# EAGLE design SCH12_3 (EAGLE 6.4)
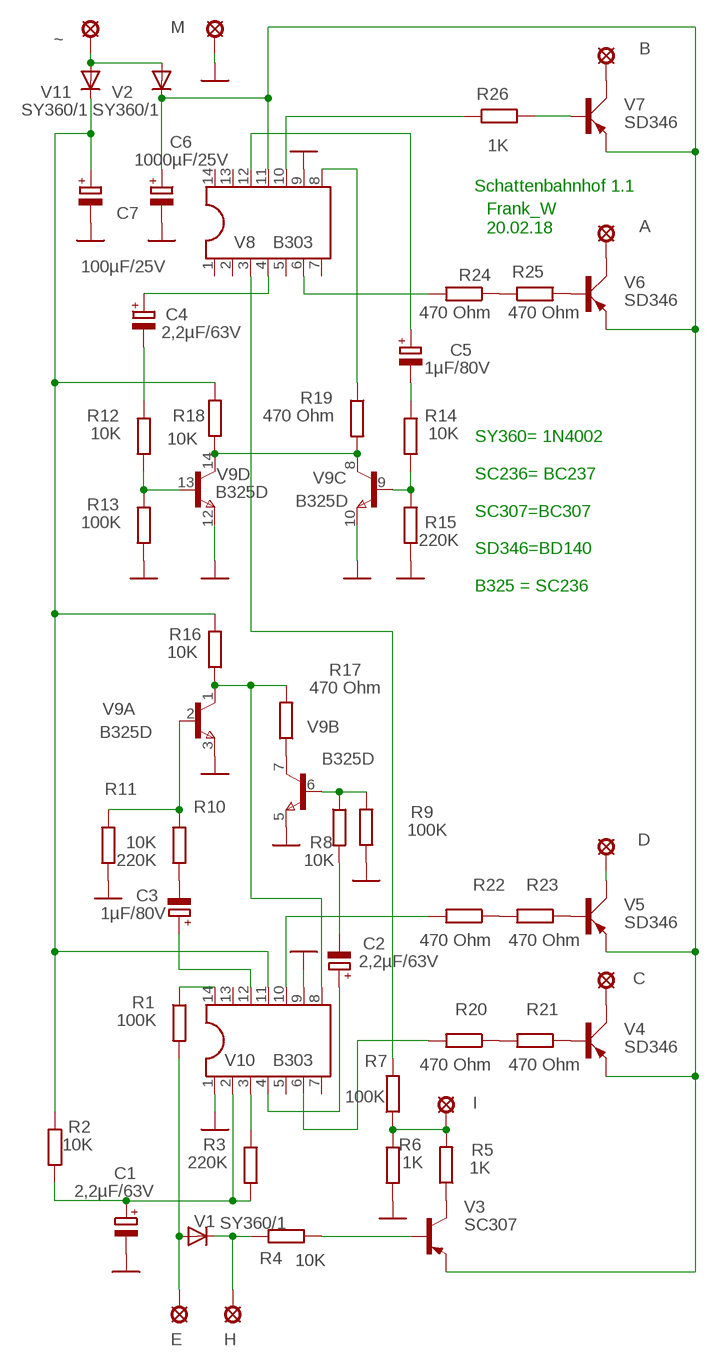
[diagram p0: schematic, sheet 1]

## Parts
A  LSP10  [LSP10]
B  LSP10  [LSP10]
C  LSP10  [LSP10]
C1  2,2µF/63V  CPOL-EUE5-5  [E5-5]
C2  2,2µF/63V  CPOL-EUE5-5  [E5-5]
C3  1µF/80V  CPOL-EUE2-5  [E2-5]
C4  2,2µF/63V  CPOL-EUE2-5  [E2-5]
C5  1µF/80V  CPOL-EUE5-5  [E5-5]
C6  1000µF/25V  CPOL-EUE22-9AXIAL  [E22-9]
C7  100µF/25V  CPOL-EUE2.5-6  [E2,5-6]
D  LSP10  [LSP10]
E  LSP10  [LSP10]
H  LSP10  [LSP10]
I  LSP10  [LSP10]
M  LSP10  [LSP10]
R1  100K  R-EU_0207/12  [0207/12]
R2  10K  R-EU_0207/12  [0207/12]
R3  220K  R-EU_0207/12  [0207/12]
R4  10K  R-EU_0207/12  [0207/12]
R5  1K  R-EU_0207/12  [0207/12]
R6  1K  R-EU_0207/12  [0207/12]
R7  100K  R-EU_0207/12  [0207/12]
R8  10K  R-EU_0207/12  [0207/12]
R9  100K  R-EU_0207/12  [0207/12]
R10  10K  R-EU_0207/12  [0207/12]
R11  220K  R-EU_0207/12  [0207/12]
R12  10K  R-EU_0207/12  [0207/12]
R13  100K  R-EU_0207/12  [0207/12]
R14  10K  R-EU_0207/12  [0207/12]
R15  220K  R-EU_0207/12  [0207/12]
R16  10K  R-EU_0207/12  [0207/12]
R17  470 Ohm  R-EU_0207/12  [0207/12]
R18  10K  R-EU_0207/12  [0207/12]
R19  470 Ohm  R-EU_0207/12  [0207/12]
R20  470 Ohm  R-EU_0207/12  [0207/12]
R21  470 Ohm  R-EU_0207/12  [0207/12]
R22  470 Ohm  R-EU_0207/12  [0207/12]
R23  470 Ohm  R-EU_0207/12  [0207/12]
R24  470 Ohm  R-EU_0207/12  [0207/12]
R25  470 Ohm  R-EU_0207/10  [0207/10]
R26  1K  R-EU_0207/10  [0207/10]
V1  SY360/1  1N4004  [DO41-10]
V2  SY360/1  1N4004  [DO41-10]
V3  SC307  BC448  [TO92-EBC]
V4  SD346  BD140  [TO126AV]
V5  SD346  BD140  [TO126AV]
V6  SD346  BD140  [TO126AV]
V7  SD346  BD140  [TO126AV]
V8  B303  DIL14  [DIL14]
V9  B325D  MAT-04Y  [DIL14]
V10  B303  DIL14  [DIL14]
V11  SY360/1  1N4004  [DO41-10]
~  LSP10  [LSP10]

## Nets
GND: C1.- C6.- C7.- M.MP R6.2 R9.1 R11.2 R13.2 R15.2 V8.9 V9.3(A:E) V9.5(B:E) V9.10(C:E) V9.12(D:E) V10.1 V10.9
N$1: V2.A V11.A ~.MP
N$2: B.MP V7.C
N$3: A.MP V6.C
N$4: R17.1 V9.7(B:C)
N$5: R25.2 V6.B
N$6: R26.2 V7.B
N$7: R19.1 V8.8
N$8: C5.+ V8.12
N$9: C5.- R14.1
N$10: R26.1 V8.10
N$11: R24.1 R25.1
N$13: C7.+ R2.1 R16.2 R18.2 V10.11 V11.C
N$14: R16.1 R17.2 V9.1(A:C) V10.8
N$15: C4.+ V8.4
N$16: C4.- R12.1
N$17: R24.2 V8.6
N$18: E.MP R1.2 V1.A
N$19: R1.1 V10.14
N$20: H.MP R4.2 V1.C
N$21: I.MP R5.2 R6.1 R7.1
N$22: R4.1 V3.B
N$23: R5.1 V3.C
N$24: C6.+ V2.C V3.E V4.E V5.E V6.E V7.E V8.11
N$25: C.MP V4.C
N$26: D.MP V5.C
N$27: R21.1 V4.B
N$28: R23.1 V5.B
N$29: C1.+ R2.2 R3.2 V10.2
N$30: C2.+ V10.4
N$31: R3.1 V10.3
N$32: C2.- R8.2
N$33: R20.2 V10.6
N$34: R8.1 R9.2 V9.6(B:B)
N$35: C3.- R10.2
N$36: C3.+ V10.12
N$37: R22.2 V10.10
N$39: R10.1 R11.1 V9.2(A:B)
N$40: R12.2 R13.1 V9.13(D:B)
N$41: R18.1 R19.2 V9.8(C:C) V9.14(D:C)
N$42: R14.2 R15.1 V9.9(C:B)
N$43: R20.1 R21.2
N$44: R22.1 R23.2
N$46: R7.2 V8.3
Unconnected: V8.1 V8.2 V8.5 V8.7 V8.13 V8.14 V10.5 V10.7 V10.13

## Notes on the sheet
- Schattenbahnhof 1.1
- Frank_W
  20.02.18
- SY360= 1N4002
  
  SC236= BC237
  
  SC307=BC307
  
  SD346=BD140
  
  B325 = SC236

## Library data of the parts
A B C D E H I M ~ = solpad:LSP10: SOLDER PAD
C1-C7 = rcl:CPOL-EU: POLARIZED CAPACITOR, European symbol
R1-R26 = rcl:R-EU_: RESISTOR, European symbol
V1 V2 V11 = diode:1N4004: DIODE
V3 = transistor-pnp:BC448*: PNP Transistror
V4-V7 = transistor-power:BD140: PNP TRANSISTOR
V8 V10 = ic-package:DIL14: Dual In Line / Socket
V9 = linear:MAT-04: Quad TRANSISTOR

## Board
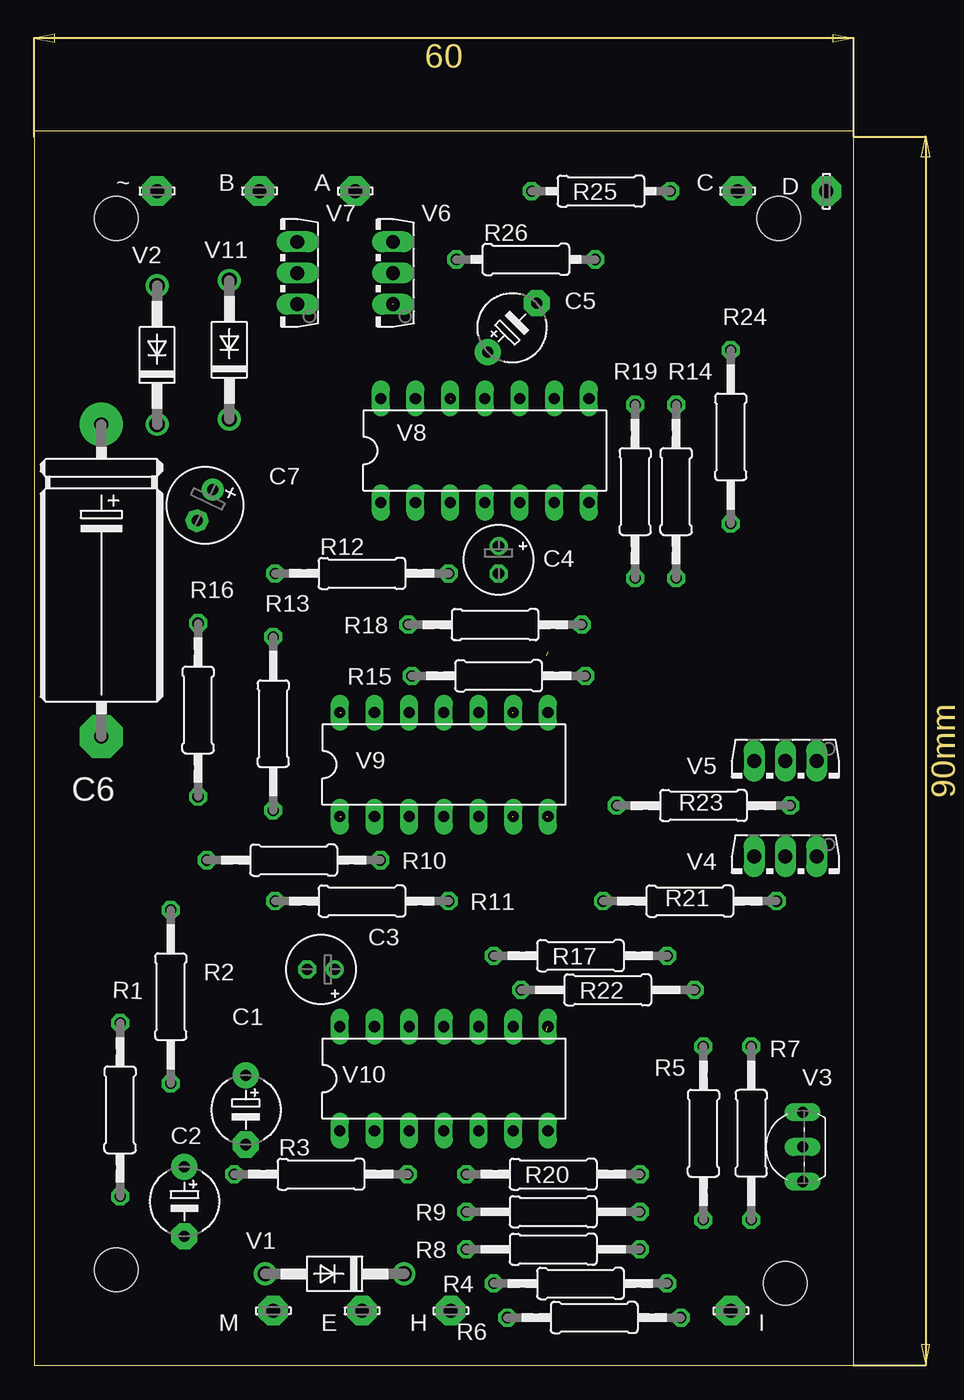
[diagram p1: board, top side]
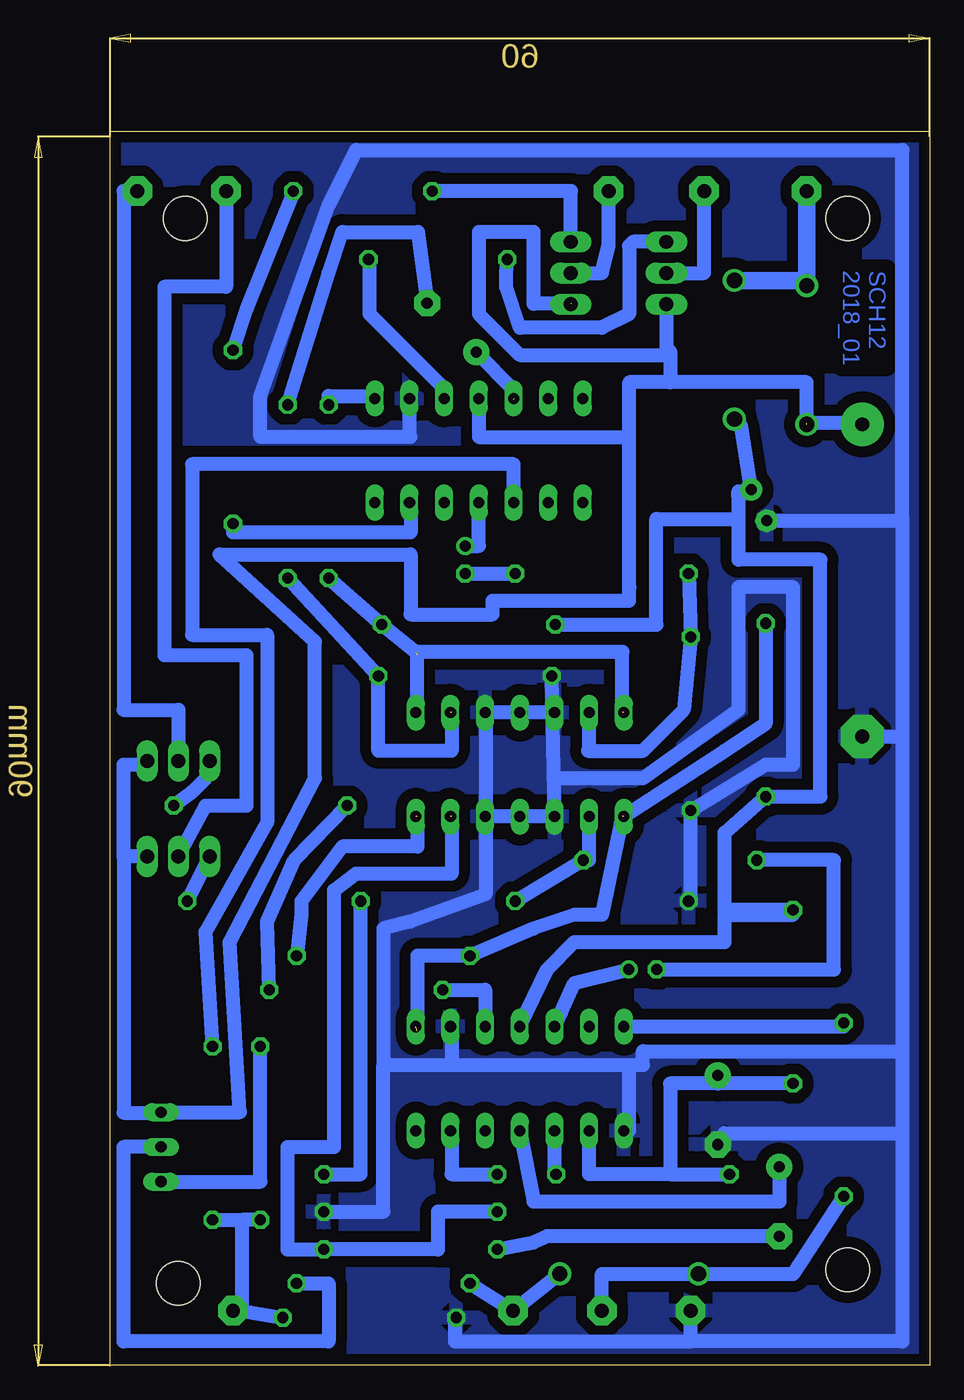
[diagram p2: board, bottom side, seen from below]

Size 65.56 x 97.5 mm. Coordinates in mm from the lower left corner, seen from the top.
Outline: 0,90.4 0,0 60,0 60,90.4 0,90.4
Copper layers (1*16): Top 0.035mm / dielectric 1.5mm / Bottom 0.035mm
Design rules "default *": minimum track width 20mil, minimum drill 24mil, track to track 8mil, track to pad 8mil, pad to pad 8mil, via to via 8mil, smd to smd 8mil, copper to edge 20mil, drill to drill 8mil, minimum pad ring 10mil, minimum via ring 8mil, stop-mask expansion 4mil, vias tented up to drill 0mil, thermal gap 20mil
Holes 3.2 mm at 55,6 6,7 6,84 54.5,84

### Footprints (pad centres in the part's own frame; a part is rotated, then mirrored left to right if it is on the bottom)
LSP10 = drill 1.016 pad 2.159 octagon: MP 0,0
E5-5 = drill 0.813 pad 1.905: + -2.54,0 | drill 0.813 pad 1.905 octagon: - 2.54,0
E2-5 = drill 0.813 pad 1.27: + -1.016,0 | drill 0.813 pad 1.27 octagon: - 1.016,0
E22-9 = drill 1.016 pad 3.15: + -11.43,0 | drill 1.016 pad 3.15 octagon: - 11.43,0
E2,5-6 = drill 0.813 pad 1.6: + -1.27,0 | drill 0.813 pad 1.6 octagon: - 1.27,0
0207/12 = drill 0.813 octagon: 1 -6.35,0; 2 6.35,0
0207/10 = drill 0.813 octagon: 1 -5.08,0; 2 5.08,0
DO41-10 = drill 1.118: A 5.08,0; C -5.08,0
TO92-EBC = drill 0.813 long: B 0,-1.27; C -2.54,-1.27; E 2.54,-1.27
TO126AV = drill 1.016 long: B 2.286,-1.27; C 0,-1.27; E -2.286,-1.27
DIL14 = drill 0.813 long: 1 -7.62,-3.81; 2 -5.08,-3.81; 3 -2.54,-3.81; 4 0,-3.81; 5 2.54,-3.81; 6 5.08,-3.81; 7 7.62,-3.81; 8 7.62,3.81; 9 5.08,3.81; 10 2.54,3.81; 11 0,3.81; 12 -2.54,3.81; 13 -5.08,3.81; 14 -7.62,3.81

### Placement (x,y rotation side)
A  23.5,86 0 top
B  16.5,86 0 top
C  51.5,86 0 top
C1  15.5,18.71 270 top
C2  11,12 270 top
C3  21,29 180 top
C4  34,59 270 top
C5  35,76 45 top
C6  4.92,57.49 270 top
C7  12.5,63 243.5 top
D  58,86 90 top
E  24,4 0 top
H  30.5,4 0 top
I  51,4 0 top
M  17.5,4 0 top
R1  6.29,18.72 270 top
R2  10,27 270 top
R3  21,14 180 top
R4  40,6 180 top
R5  49,17 270 top
R6  41,3.5 180 top
R7  52.5,17 90 top
R8  38,8.5 180 top
R9  38,11.25 180 top
R10  19,37 180 top
R11  24,34 180 top
R12  24,58 180 top
R13  17.5,47 270 top
R14  47,64 270 top
R15  34,50.5 180 top
R16  12,48 270 top
R17  40,30 180 top
R18  33.75,54.25 180 top
R19  44,64 270 top
R20  38,14 180 top
R21  48,34 180 top
R22  42,27.5 180 top
R23  49,41 180 top
R24  51,68 270 top
R25  41.5,86 180 top
R26  36,81 180 top
V1  22,6.7 180 top
V2  9,74 90 top
V3  55,16 90 top
V4  55,36 180 top
V5  55,43 180 top
V6  25,80 90 top
V7  18,80 90 top
V8  33,67 0 top
V9  30,44 0 top
V10  30,21 0 top
V11  14.29,74.38 90 top
~  9,86 0 top

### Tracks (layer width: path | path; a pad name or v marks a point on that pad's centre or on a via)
GND
  Bottom 1.016: C7.- 2,61.86 2,46.06 | 2,62 2,89 42,89 44,85 49,71 49,68 38,68 38.08,68.08 V8.9 | 2,46.06 2,23 | 2,23 2,17 | 2,17 2,1.75 17.5,1.75 | 17.5,1.75 M.MP | C1.- 15,16.17 15,17 2,17 | C6.- 2,46.06 | 34.75,3.5 34.75,1.75 17.5,1.75 | V10.9 35,24.81 35,22 | 35,22 22,22 | 22,22 21,22 21,23 2,23 | R9.1 40,11.25 40,22 | 40,22 35,22 | 32.5,47.81 32.5,40.19 | 32.5,40.19 32.5,34.5 38,32.5 40,32 40,22 | 27.46,43 21,43 14,48 14,57 10,57 10,44 12,44 R13.2 17.5,34 R11.2 | V10.1 22,17.19 22,22 | R15.2 V9.3 32.5,40.19 | V9.12 V9.10 | 32.5,40.19 V9.5
  pour Bottom (isolate 0.813): 0,90 60,90 60,0 0,0
N$1
  Bottom 1.27: V11.A 9,79.46 V2.A ~.MP
N$2
  Bottom 1.016: V7.C 16.5,80 B.MP
N$3
  Bottom 1.016: V6.C 24,80 23.5,82 A.MP
N$4  (1 unrouted)
  Bottom 1.016: 37.5,40.19 37.5,38 43,38 46,34 46,33 R17.1
N$5
  Bottom 1.016: V6.B 26.27,86 R25.2
N$6
  Bottom 1.016: V7.B 21.71,82.29 22,82 22,77 24,76 30,76 31,79 31,80 R26.2
N$7
  Bottom 1.016: R19.1 44,71 40.81,71 V8.8
N$8  (1 unrouted)
  Bottom 1.016: C5.+ 30.5,71.46 30.5,70.75
N$9
  Bottom 1.016: R14.1 44,80 43,83 37.46,83 C5.-
N$10
  Bottom 1.016: V8.10 35.54,71.54 41,77 41,81 R26.1
N$11
  Bottom 1.016: R24.1 50,77.35 46.5,86 R25.1
N$13
  Bottom 1.016: V11.C 13.79,68.8 C7.+ 14,63.59 | 14,63.59 14,64 | 14,63.59 14,62 | 14,62 14,59 8,59 8,41.65 R16.2 15,39 15,33.35 R2.1 10,33 15,33 15,31 26,31 28,29 V10.11 | R18.2 20,54.25 20,62 14,62
N$14  (2 unrouted)
  Bottom 1.016: 22.5,40.19 24,33 26,33 29,32 R17.2 37.5,30 37.5,24.5 | R16.1 12,47 15,45 V9.1
N$15
  Bottom 1.016: C4.+ 33,60.02 V8.4
N$16
  Bottom 1.016: C4.- 30.35,57.98 R12.1
N$17
  Bottom 1.016: V8.6 38,63.19 38,61 51,61 R24.2
N$18
  Bottom 1.016: E.MP 24,6.7 V1.A 10,6.7 R1.2
N$19
  Bottom 1.016: V10.14 6.29,24.81 R1.1
N$20
  Bottom 1.016: V1.C H.MP R4.2
N$21
  Bottom 1.016: R7.1 50.35,10.65 | 50.35,10.65 50.35,4 | 50.35,4 R6.1 | I.MP 50.35,4 | R5.2 50.35,10.65
N$22
  Bottom 1.016: R4.1 44,6 44,1.75 59,1.75 59,16 V3.B
N$23
  Bottom 1.016: R5.1 49,13.46 V3.C
N$24  (2 unrouted)
  Bottom 1.016: 59,37.27 59,44 57.29,44 V5.E | V7.E 19.27,74.27 | 19.27,74.27 19,74 30,74 33,77 33,83 29,83 29,77.75 26.25,77.75 | V6.E 26.71,77.71 | 9,69 9,72 19,72 | 19,72 21.98,72 | V8.11 33,68 22,68 21.98,72 | C6.+ 5,69 8.92,69 V2.C | 19.27,74.27 19,74.27 19,72 | 21.98,72 21.98,57 22,57 22,56 32,56 32,55 38,55 38,59.4 52,59.4 45,53 45,43 51.25,31 50.5,18.54 V3.E 56.27,18.5 59,18.5 59,37.27 | V4.E 59,37.27
N$25
  Bottom 1.016: C.MP 51.5,79 56,79 56,52 50,52 50,41 53,41 V4.C
N$26
  Bottom 1.016: D.MP 59,86 59,48 55,48 V5.C
N$27
  Bottom 1.016: R21.1 V4.B
N$28
  Bottom 1.016: V5.B 53,43 54,42 R23.1
N$29
  Bottom 1.016: R2.2 15.5,20.65 | 15.5,20.65 C1.+ | 15.5,20.65 19,20.65 19,14 | 19,14 R3.2 | 19,14 24.92,14 V10.2
N$30
  Bottom 1.016: V10.4 29,12 11,12 C2.+
N$31
  Bottom 1.016: R3.1 27.46,14 V10.3
N$32
  Bottom 1.016: C2.- 28,9.46 29,9 R8.2
N$33
  Bottom 1.016: V10.6 35,17.19 35,14 R20.2
N$34  (1 unrouted)
  Bottom 1.016: R9.2 36,11.25 36,8.5 R8.1 47,8.5 47,16 43.6,16 43.6,34.8 42,36 35,36 35,40.19
N$35
  Bottom 1.016: 20,29 C3.- 7,29 7,37 R10.2
N$36
  Bottom 1.016: V10.12 27,25.81 26,28 C3.+
N$37
  Bottom 1.016: R22.2 32.54,27.5 V10.10
N$39
  Bottom 1.016: R11.1 R10.1 24.92,37 V9.2
N$40
  Bottom 1.016: 24.92,45 21,45 18,48 R13.1 R12.2 | 25,45 24.92,45 | 24.92,45 V9.13
N$41  (2 unrouted)
  Bottom 1.016: 22.5,47.81 22.5,52.25 37.62,52.25 R18.1 R19.2 | V9.8 37.5,47.81 37.5,52
N$42  (1 unrouted)
  Bottom 1.016: R14.2 R15.1 40.35,45 35,45 35,47.81
N$43
  Bottom 1.016: R20.1 41.65,14 R21.2
N$44
  Bottom 1.016: R23.2 46.5,37 48.5,32.5 R22.1
N$46
  Bottom 1.016: V8.3 30.46,66 54,66 54,53.5 48.5,53.5 48.5,39.75 53,31.75 R7.2

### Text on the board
Bottom: SCH12 / 2018_01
